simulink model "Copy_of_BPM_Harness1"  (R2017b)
settings: Solver=FixedStepDiscrete  StartTime=0.0  StopTime=4  FixedStep=0.01  RelTol=1e-3  EnableMultiTasking=on
undefined symbols (not defined in the file): sigbuilder_block

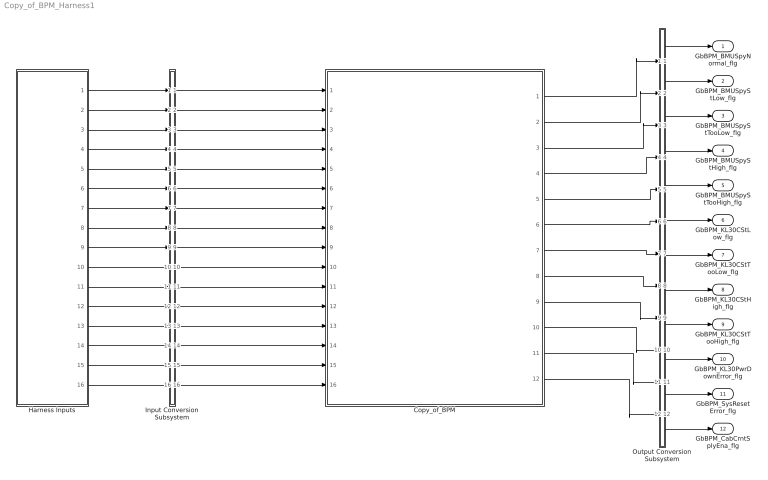
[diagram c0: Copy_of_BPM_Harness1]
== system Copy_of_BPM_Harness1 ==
  Copy_of_BPM : ModelReference  ModelNameDialog=Copy_of_BPM  SimulationMode=Normal  ModelReferenceVersion='M105C104'
  Harness Inputs : Subsystem  Tag=STV Subsys  LoadFcn=sigbuilder_block('load');  StartFcn=sigbuilder_block('start');  StopFcn=sigbuilder_block('stop');  ClipboardFcn=sigbuilder_block('clipboard');  mask(Sigbuilder block){tuvar=[0:10]}
      mask init:
      | if ~strcmp(get_param(bdroot(gcb),'SimulationStatus'),'stopped'),tuvar = sigbuilder_block('maskInit'); end
  Input Conversion Subsystem : Subsystem  Tag=__SLT_ICS__  Description=Signal spec. and routing
  Output Conversion Subsystem : Subsystem  Tag=__SLT_OCS__  Description=Signal spec. and routing
  GbBPM_BMUSpyNormal_flg : Outport  OutDataTypeStr=boolean  PortDimensions=[1]
  GbBPM_BMUSpyStLow_flg : Outport  Port=2  OutDataTypeStr=boolean  PortDimensions=[1]
  GbBPM_BMUSpyStTooLow_flg : Outport  Port=3  OutDataTypeStr=boolean  PortDimensions=[1]
  GbBPM_BMUSpyStHigh_flg : Outport  Port=4  OutDataTypeStr=boolean  PortDimensions=[1]
  GbBPM_BMUSpyStTooHigh_flg : Outport  Port=5  OutDataTypeStr=boolean  PortDimensions=[1]
  GbBPM_KL30CStLow_flg : Outport  Port=6  OutDataTypeStr=boolean  PortDimensions=[1]
  GbBPM_KL30CStTooLow_flg : Outport  Port=7  OutDataTypeStr=boolean  PortDimensions=[1]
  GbBPM_KL30CStHigh_flg : Outport  Port=8  OutDataTypeStr=boolean  PortDimensions=[1]
  GbBPM_KL30CStTooHigh_flg : Outport  Port=9  OutDataTypeStr=boolean  PortDimensions=[1]
  GbBPM_KL30PwrDownError_flg : Outport  Port=10  OutDataTypeStr=boolean  PortDimensions=[1]
  GbBPM_SysResetError_flg : Outport  Port=11  OutDataTypeStr=boolean  PortDimensions=[1]
  GbBPM_CabCrntSplyEna_flg : Outport  Port=12  OutDataTypeStr=boolean  PortDimensions=[1]
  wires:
  Harness Inputs/1(GcLDP_BmuSplyVolt_mV) -> Input Conversion Subsystem/1(Inport_1)
  Harness Inputs/2(GcLDP_Kl30CVolt_mV) -> Input Conversion Subsystem/2(Inport_2)
  Harness Inputs/3(GbISP_TFBMUSpyStLow_flg) -> Input Conversion Subsystem/3(Inport_3)
  Harness Inputs/4(GbISP_TFBMUSpyStTooLow_flg) -> Input Conversion Subsystem/4(Inport_4)
  Harness Inputs/5(GbISP_TFBMUSpyStHigh_flg) -> Input Conversion Subsystem/5(Inport_5)
  Harness Inputs/6(GbISP_TFBMUSpyStTooHigh_flg) -> Input Conversion Subsystem/6(Inport_6)
  Harness Inputs/7(GbISP_TFKL30CStLow_flg) -> Input Conversion Subsystem/7(Inport_7)
  Harness Inputs/8(GbISP_TFKL30CStTooLow_flg) -> Input Conversion Subsystem/8(Inport_8)
  Harness Inputs/9(GbISP_TFKL30CStHigh_flg) -> Input Conversion Subsystem/9(Inport_9)
  Harness Inputs/10(GbISP_TFKL30CStTooHigh_flg) -> Input Conversion Subsystem/10(Inport_10)
  Harness Inputs/11(GeMSM_BMUState_enum) -> Input Conversion Subsystem/11(Inport_11)
  Harness Inputs/12(GeISP_BMULastPwrDown_enum) -> Input Conversion Subsystem/12(Inport_12)
  Harness Inputs/13(GeISP_BMULastReset_enum) -> Input Conversion Subsystem/13(Inport_13)
  Harness Inputs/14(GeISP_NetWkUpSt_enum) -> Input Conversion Subsystem/14(Inport_14)
  Harness Inputs/15(GcLDP_Kl30Volt_mV) -> Input Conversion Subsystem/15(Inport_15)
  Harness Inputs/16(GeISP_DiagComSt_enum) -> Input Conversion Subsystem/16(Inport_16)
  Output Conversion Subsystem/1(Outport_1) -> GbBPM_BMUSpyNormal_flg/1
  Output Conversion Subsystem/2(Outport_2) -> GbBPM_BMUSpyStLow_flg/1
  Output Conversion Subsystem/3(Outport_3) -> GbBPM_BMUSpyStTooLow_flg/1
  Output Conversion Subsystem/4(Outport_4) -> GbBPM_BMUSpyStHigh_flg/1
  Output Conversion Subsystem/5(Outport_5) -> GbBPM_BMUSpyStTooHigh_flg/1
  Output Conversion Subsystem/6(Outport_6) -> GbBPM_KL30CStLow_flg/1
  Output Conversion Subsystem/7(Outport_7) -> GbBPM_KL30CStTooLow_flg/1
  Output Conversion Subsystem/8(Outport_8) -> GbBPM_KL30CStHigh_flg/1
  Output Conversion Subsystem/9(Outport_9) -> GbBPM_KL30CStTooHigh_flg/1
  Output Conversion Subsystem/10(Outport_10) -> GbBPM_KL30PwrDownError_flg/1
  Output Conversion Subsystem/11(Outport_11) -> GbBPM_SysResetError_flg/1
  Output Conversion Subsystem/12(Outport_12) -> GbBPM_CabCrntSplyEna_flg/1
  Input Conversion Subsystem/1(Outport_1) -> Copy_of_BPM/1
  Input Conversion Subsystem/2(Outport_2) -> Copy_of_BPM/2
  Input Conversion Subsystem/3(Outport_3) -> Copy_of_BPM/3
  Input Conversion Subsystem/4(Outport_4) -> Copy_of_BPM/4
  Input Conversion Subsystem/5(Outport_5) -> Copy_of_BPM/5
  Input Conversion Subsystem/6(Outport_6) -> Copy_of_BPM/6
  Input Conversion Subsystem/7(Outport_7) -> Copy_of_BPM/7
  Input Conversion Subsystem/8(Outport_8) -> Copy_of_BPM/8
  Input Conversion Subsystem/9(Outport_9) -> Copy_of_BPM/9
  Input Conversion Subsystem/10(Outport_10) -> Copy_of_BPM/10
  Input Conversion Subsystem/11(Outport_11) -> Copy_of_BPM/11
  Input Conversion Subsystem/12(Outport_12) -> Copy_of_BPM/12
  Input Conversion Subsystem/13(Outport_13) -> Copy_of_BPM/13
  Input Conversion Subsystem/14(Outport_14) -> Copy_of_BPM/14
  Input Conversion Subsystem/15(Outport_15) -> Copy_of_BPM/15
  Input Conversion Subsystem/16(Outport_16) -> Copy_of_BPM/16
  Copy_of_BPM/1 -> Output Conversion Subsystem/1(Inport_1)
  Copy_of_BPM/2 -> Output Conversion Subsystem/2(Inport_2)
  Copy_of_BPM/3 -> Output Conversion Subsystem/3(Inport_3)
  Copy_of_BPM/4 -> Output Conversion Subsystem/4(Inport_4)
  Copy_of_BPM/5 -> Output Conversion Subsystem/5(Inport_5)
  Copy_of_BPM/6 -> Output Conversion Subsystem/6(Inport_6)
  Copy_of_BPM/7 -> Output Conversion Subsystem/7(Inport_7)
  Copy_of_BPM/8 -> Output Conversion Subsystem/8(Inport_8)
  Copy_of_BPM/9 -> Output Conversion Subsystem/9(Inport_9)
  Copy_of_BPM/10 -> Output Conversion Subsystem/10(Inport_10)
  Copy_of_BPM/11 -> Output Conversion Subsystem/11(Inport_11)
  Copy_of_BPM/12 -> Output Conversion Subsystem/12(Inport_12)

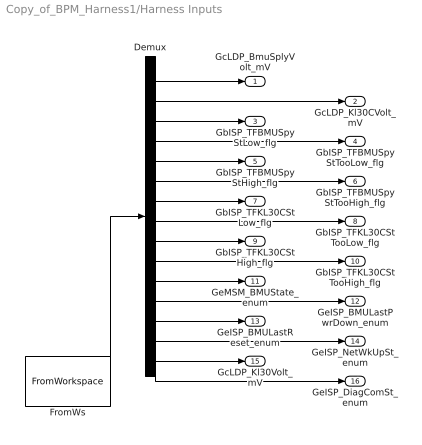
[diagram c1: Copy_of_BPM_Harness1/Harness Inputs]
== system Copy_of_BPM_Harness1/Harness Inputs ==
  Demux : Demux  Tag=STV Demux  Outputs=16
  FromWs : FromWorkspace  Tag=STV FromWs  VariableName=tuvar  SampleTime=0
  GcLDP_BmuSplyVolt_mV : Outport  Tag=STV Outport
  GcLDP_Kl30CVolt_mV : Outport  Tag=STV Outport  Port=2
  GbISP_TFBMUSpyStLow_flg : Outport  Tag=STV Outport  Port=3
  GbISP_TFBMUSpyStTooLow_flg : Outport  Tag=STV Outport  Port=4
  GbISP_TFBMUSpyStHigh_flg : Outport  Tag=STV Outport  Port=5
  GbISP_TFBMUSpyStTooHigh_flg : Outport  Tag=STV Outport  Port=6
  GbISP_TFKL30CStLow_flg : Outport  Tag=STV Outport  Port=7
  GbISP_TFKL30CStTooLow_flg : Outport  Tag=STV Outport  Port=8
  GbISP_TFKL30CStHigh_flg : Outport  Tag=STV Outport  Port=9
  GbISP_TFKL30CStTooHigh_flg : Outport  Tag=STV Outport  Port=10
  GeMSM_BMUState_enum : Outport  Tag=STV Outport  Port=11
  GeISP_BMULastPwrDown_enum : Outport  Tag=STV Outport  Port=12
  GeISP_BMULastReset_enum : Outport  Tag=STV Outport  Port=13
  GeISP_NetWkUpSt_enum : Outport  Tag=STV Outport  Port=14
  GcLDP_Kl30Volt_mV : Outport  Tag=STV Outport  Port=15
  GeISP_DiagComSt_enum : Outport  Tag=STV Outport  Port=16
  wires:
  FromWs/1 -> Demux/1
  Demux/1 -> GcLDP_BmuSplyVolt_mV/1
  Demux/2 -> GcLDP_Kl30CVolt_mV/1
  Demux/3 -> GbISP_TFBMUSpyStLow_flg/1
  Demux/4 -> GbISP_TFBMUSpyStTooLow_flg/1
  Demux/5 -> GbISP_TFBMUSpyStHigh_flg/1
  Demux/6 -> GbISP_TFBMUSpyStTooHigh_flg/1
  Demux/7 -> GbISP_TFKL30CStLow_flg/1
  Demux/8 -> GbISP_TFKL30CStTooLow_flg/1
  Demux/9 -> GbISP_TFKL30CStHigh_flg/1
  Demux/10 -> GbISP_TFKL30CStTooHigh_flg/1
  Demux/11 -> GeMSM_BMUState_enum/1
  Demux/12 -> GeISP_BMULastPwrDown_enum/1
  Demux/13 -> GeISP_BMULastReset_enum/1
  Demux/14 -> GeISP_NetWkUpSt_enum/1
  Demux/15 -> GcLDP_Kl30Volt_mV/1
  Demux/16 -> GeISP_DiagComSt_enum/1

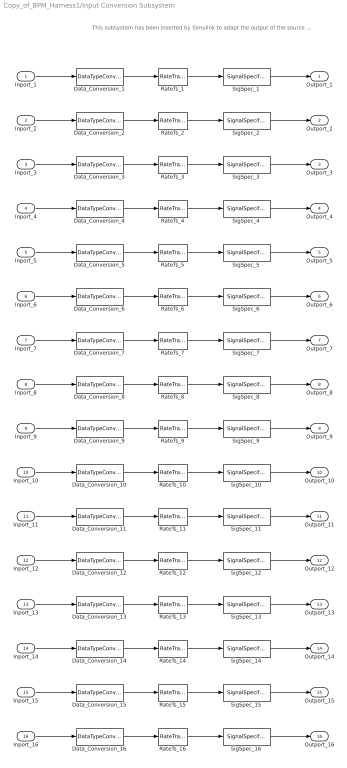
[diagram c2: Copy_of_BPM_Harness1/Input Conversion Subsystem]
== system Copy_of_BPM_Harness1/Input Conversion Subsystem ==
  note: This subsystem has been inserted by Simulink to adapt the output of the source blocks to the interface required by the harnessed component. Modifying the contents of this subsystem may result in compilation and simulation failure.
  Inport_1 : Inport
  Inport_2 : Inport  Port=2
  Inport_3 : Inport  Port=3
  Inport_4 : Inport  Port=4
  Inport_5 : Inport  Port=5
  Inport_6 : Inport  Port=6
  Inport_7 : Inport  Port=7
  Inport_8 : Inport  Port=8
  Inport_9 : Inport  Port=9
  Inport_10 : Inport  Port=10
  Inport_11 : Inport  Port=11
  Inport_12 : Inport  Port=12
  Inport_13 : Inport  Port=13
  Inport_14 : Inport  Port=14
  Inport_15 : Inport  Port=15
  Inport_16 : Inport  Port=16
  Data_Conversion_1 : DataTypeConversion  OutDataTypeStr=uint16
  Data_Conversion_{3..10} (8 alike) : DataTypeConversion  OutDataTypeStr=boolean
  Data_Conversion_{11..14,16} (5 alike) : DataTypeConversion  OutDataTypeStr=uint8
  Data_Conversion_15 : DataTypeConversion  OutDataTypeStr=uint16
  Data_Conversion_2 : DataTypeConversion  OutDataTypeStr=uint16
  RateTs_{1..16} (16 alike) : RateTransition  OutPortSampleTime=0.01
  SigSpec_1 : SignalSpecification  OutDataTypeStr=uint16  Unit=V  Dimensions=[1]  SampleTime=0.01
  SigSpec_{3..10} (8 alike) : SignalSpecification  OutDataTypeStr=boolean  Unit=flag  Dimensions=[1]  SampleTime=0.01
  SigSpec_{11..14,16} (5 alike) : SignalSpecification  OutDataTypeStr=uint8  Unit=enum  Dimensions=[1]  SampleTime=0.01
  SigSpec_15 : SignalSpecification  OutDataTypeStr=uint16  Unit=mv  Dimensions=[1]  SampleTime=0.01
  SigSpec_2 : SignalSpecification  OutDataTypeStr=uint16  Unit=mv  Dimensions=[1]  SampleTime=0.01
  Outport_1 : Outport
  Outport_2 : Outport  Port=2
  Outport_3 : Outport  Port=3
  Outport_4 : Outport  Port=4
  Outport_5 : Outport  Port=5
  Outport_6 : Outport  Port=6
  Outport_7 : Outport  Port=7
  Outport_8 : Outport  Port=8
  Outport_9 : Outport  Port=9
  Outport_10 : Outport  Port=10
  Outport_11 : Outport  Port=11
  Outport_12 : Outport  Port=12
  Outport_13 : Outport  Port=13
  Outport_14 : Outport  Port=14
  Outport_15 : Outport  Port=15
  Outport_16 : Outport  Port=16
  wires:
  SigSpec_1/1 -> Outport_1/1
  RateTs_1/1 -> SigSpec_1/1
  Data_Conversion_1/1 -> RateTs_1/1
  Inport_1/1 -> Data_Conversion_1/1
  SigSpec_2/1 -> Outport_2/1
  RateTs_2/1 -> SigSpec_2/1
  Data_Conversion_2/1 -> RateTs_2/1
  Inport_2/1 -> Data_Conversion_2/1
  SigSpec_3/1 -> Outport_3/1
  RateTs_3/1 -> SigSpec_3/1
  Data_Conversion_3/1 -> RateTs_3/1
  Inport_3/1 -> Data_Conversion_3/1
  SigSpec_4/1 -> Outport_4/1
  RateTs_4/1 -> SigSpec_4/1
  Data_Conversion_4/1 -> RateTs_4/1
  Inport_4/1 -> Data_Conversion_4/1
  SigSpec_5/1 -> Outport_5/1
  RateTs_5/1 -> SigSpec_5/1
  Data_Conversion_5/1 -> RateTs_5/1
  Inport_5/1 -> Data_Conversion_5/1
  SigSpec_6/1 -> Outport_6/1
  RateTs_6/1 -> SigSpec_6/1
  Data_Conversion_6/1 -> RateTs_6/1
  Inport_6/1 -> Data_Conversion_6/1
  SigSpec_7/1 -> Outport_7/1
  RateTs_7/1 -> SigSpec_7/1
  Data_Conversion_7/1 -> RateTs_7/1
  Inport_7/1 -> Data_Conversion_7/1
  SigSpec_8/1 -> Outport_8/1
  RateTs_8/1 -> SigSpec_8/1
  Data_Conversion_8/1 -> RateTs_8/1
  Inport_8/1 -> Data_Conversion_8/1
  SigSpec_9/1 -> Outport_9/1
  RateTs_9/1 -> SigSpec_9/1
  Data_Conversion_9/1 -> RateTs_9/1
  Inport_9/1 -> Data_Conversion_9/1
  SigSpec_10/1 -> Outport_10/1
  RateTs_10/1 -> SigSpec_10/1
  Data_Conversion_10/1 -> RateTs_10/1
  Inport_10/1 -> Data_Conversion_10/1
  SigSpec_11/1 -> Outport_11/1
  RateTs_11/1 -> SigSpec_11/1
  Data_Conversion_11/1 -> RateTs_11/1
  Inport_11/1 -> Data_Conversion_11/1
  SigSpec_12/1 -> Outport_12/1
  RateTs_12/1 -> SigSpec_12/1
  Data_Conversion_12/1 -> RateTs_12/1
  Inport_12/1 -> Data_Conversion_12/1
  SigSpec_13/1 -> Outport_13/1
  RateTs_13/1 -> SigSpec_13/1
  Data_Conversion_13/1 -> RateTs_13/1
  Inport_13/1 -> Data_Conversion_13/1
  SigSpec_14/1 -> Outport_14/1
  RateTs_14/1 -> SigSpec_14/1
  Data_Conversion_14/1 -> RateTs_14/1
  Inport_14/1 -> Data_Conversion_14/1
  SigSpec_15/1 -> Outport_15/1
  RateTs_15/1 -> SigSpec_15/1
  Data_Conversion_15/1 -> RateTs_15/1
  Inport_15/1 -> Data_Conversion_15/1
  SigSpec_16/1 -> Outport_16/1
  RateTs_16/1 -> SigSpec_16/1
  Data_Conversion_16/1 -> RateTs_16/1
  Inport_16/1 -> Data_Conversion_16/1

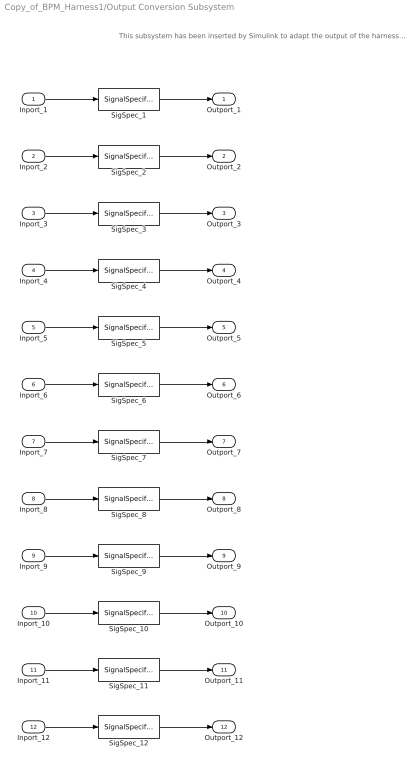
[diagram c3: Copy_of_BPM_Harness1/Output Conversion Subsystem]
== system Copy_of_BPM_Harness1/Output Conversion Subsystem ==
  note: This subsystem has been inserted by Simulink to adapt the output of the harnessed component to the interface required by the sink blocks. Modifying the contents of this subsystem may result in compilation and simulation failure.
  Inport_1 : Inport
  Inport_2 : Inport  Port=2
  Inport_3 : Inport  Port=3
  Inport_4 : Inport  Port=4
  Inport_5 : Inport  Port=5
  Inport_6 : Inport  Port=6
  Inport_7 : Inport  Port=7
  Inport_8 : Inport  Port=8
  Inport_9 : Inport  Port=9
  Inport_10 : Inport  Port=10
  Inport_11 : Inport  Port=11
  Inport_12 : Inport  Port=12
  SigSpec_1 : SignalSpecification  OutDataTypeStr=boolean  Unit=flg  Dimensions=[1]  SampleTime=0.01
  SigSpec_{2..11} (10 alike) : SignalSpecification  OutDataTypeStr=boolean  Unit=flag  Dimensions=[1]  SampleTime=0.01
  SigSpec_12 : SignalSpecification  OutDataTypeStr=boolean  Unit=flg  Dimensions=[1]  SampleTime=0.01
  Outport_1 : Outport
  Outport_2 : Outport  Port=2
  Outport_3 : Outport  Port=3
  Outport_4 : Outport  Port=4
  Outport_5 : Outport  Port=5
  Outport_6 : Outport  Port=6
  Outport_7 : Outport  Port=7
  Outport_8 : Outport  Port=8
  Outport_9 : Outport  Port=9
  Outport_10 : Outport  Port=10
  Outport_11 : Outport  Port=11
  Outport_12 : Outport  Port=12
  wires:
  Inport_1/1 -> SigSpec_1/1
  SigSpec_1/1 -> Outport_1/1
  Inport_2/1 -> SigSpec_2/1
  SigSpec_2/1 -> Outport_2/1
  Inport_3/1 -> SigSpec_3/1
  SigSpec_3/1 -> Outport_3/1
  Inport_4/1 -> SigSpec_4/1
  SigSpec_4/1 -> Outport_4/1
  Inport_5/1 -> SigSpec_5/1
  SigSpec_5/1 -> Outport_5/1
  Inport_6/1 -> SigSpec_6/1
  SigSpec_6/1 -> Outport_6/1
  Inport_7/1 -> SigSpec_7/1
  SigSpec_7/1 -> Outport_7/1
  Inport_8/1 -> SigSpec_8/1
  SigSpec_8/1 -> Outport_8/1
  Inport_9/1 -> SigSpec_9/1
  SigSpec_9/1 -> Outport_9/1
  Inport_10/1 -> SigSpec_10/1
  SigSpec_10/1 -> Outport_10/1
  Inport_11/1 -> SigSpec_11/1
  SigSpec_11/1 -> Outport_11/1
  Inport_12/1 -> SigSpec_12/1
  SigSpec_12/1 -> Outport_12/1
